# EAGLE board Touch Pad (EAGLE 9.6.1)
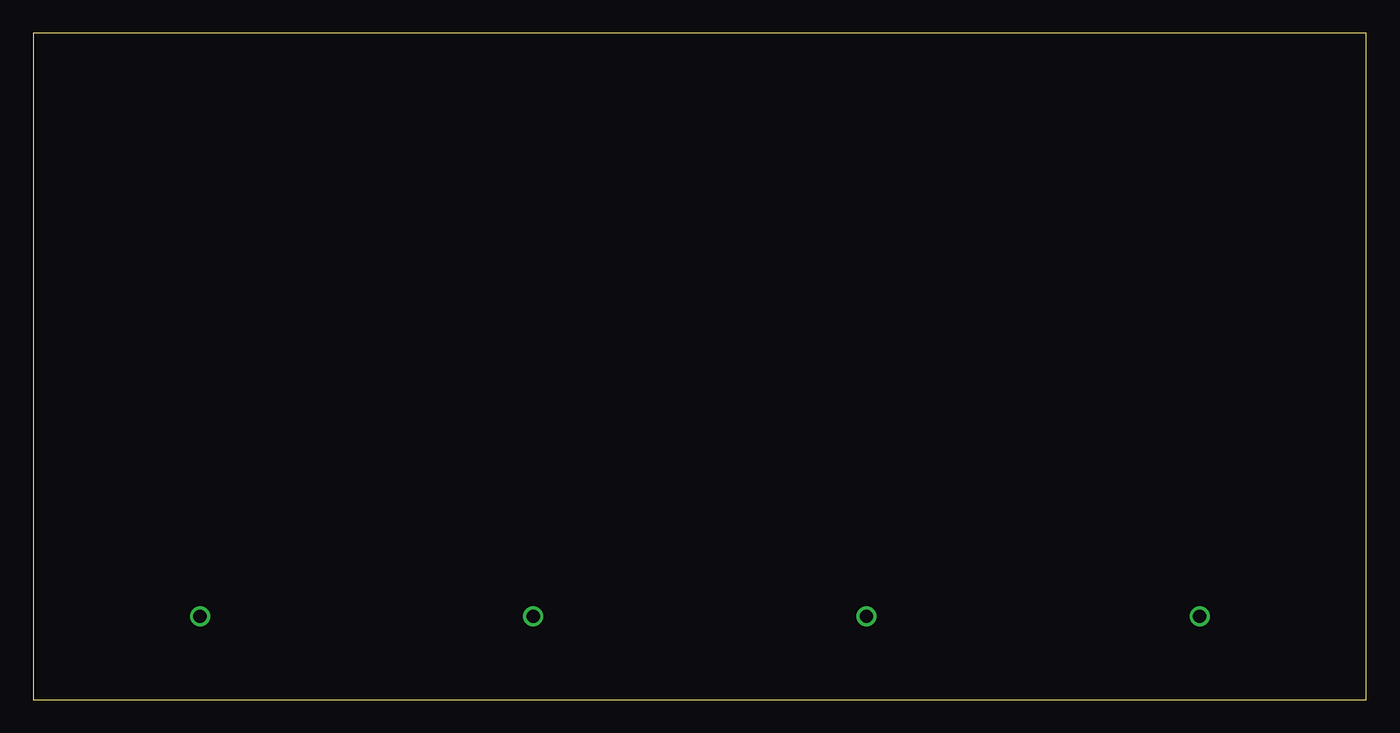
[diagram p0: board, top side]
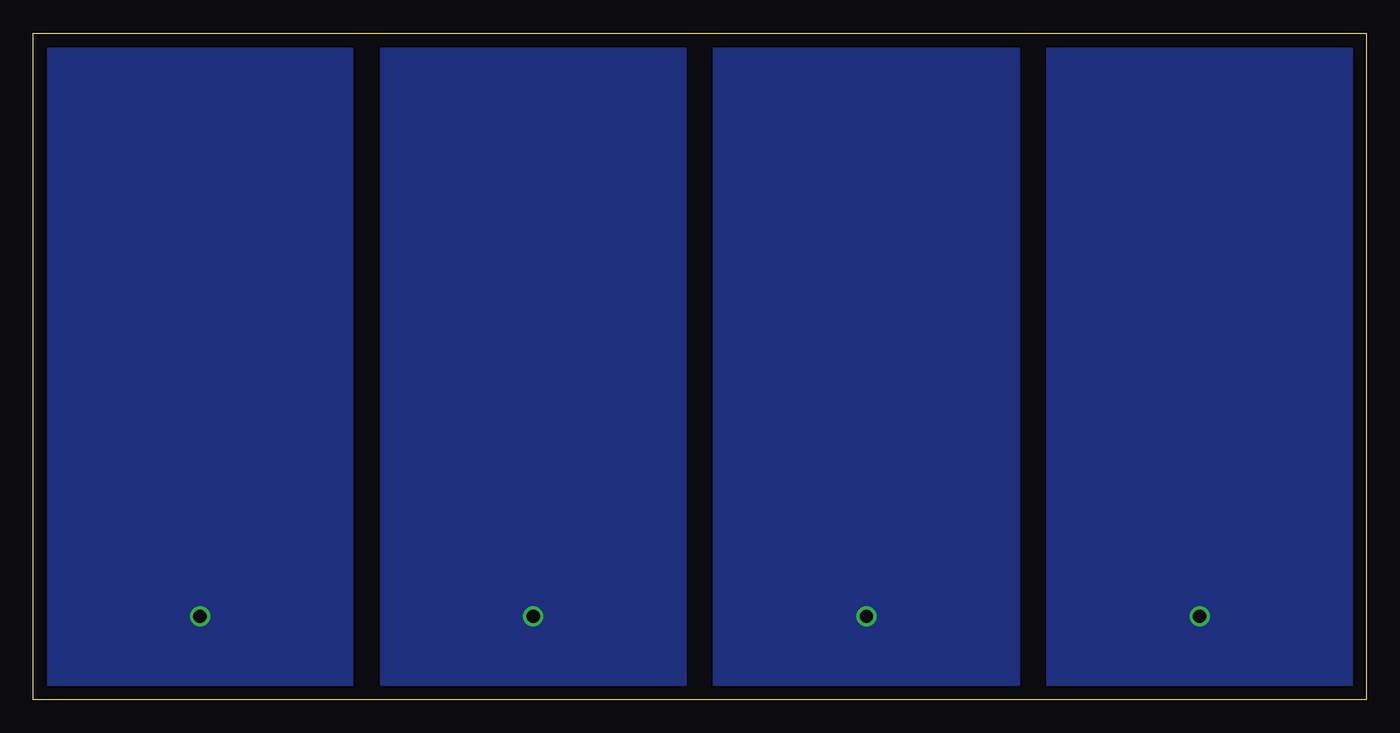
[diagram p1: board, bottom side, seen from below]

Size 100 x 50 mm. Coordinates in mm from the lower left corner, seen from the top.
Outline: 100,0 100,50 0,50 0,0 100,0
Copper layers (1*16): Top 0.035mm / dielectric 1.5mm / Bottom 0.035mm
Design rules "default": minimum track width 6mil, minimum drill 0.35mm, track to track 6mil, track to pad 6mil, pad to pad 6mil, via to via 6mil, smd to smd 6mil, copper to edge 40mil, drill to drill 6mil, minimum pad ring 10mil, minimum via ring 8mil, stop-mask expansion 4mil, vias tented up to drill 0mil, thermal gap 10mil

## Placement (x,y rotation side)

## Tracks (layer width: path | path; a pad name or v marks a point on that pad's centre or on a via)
N$1  (via drill 1)
  other vias: 12.5,6.25
  pour Bottom: 1,1 1,49 24,49 24,1
N$2  (via drill 1)
  other vias: 37.5,6.25
  pour Bottom: 26,1 26,49 49,49 49,1
N$3  (via drill 1)
  other vias: 62.5,6.25
  pour Bottom: 51,1 51,49 74,49 74,1
N$4  (via drill 1)
  other vias: 87.5,6.25
  pour Bottom: 76,1 76,49 99,49 99,1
